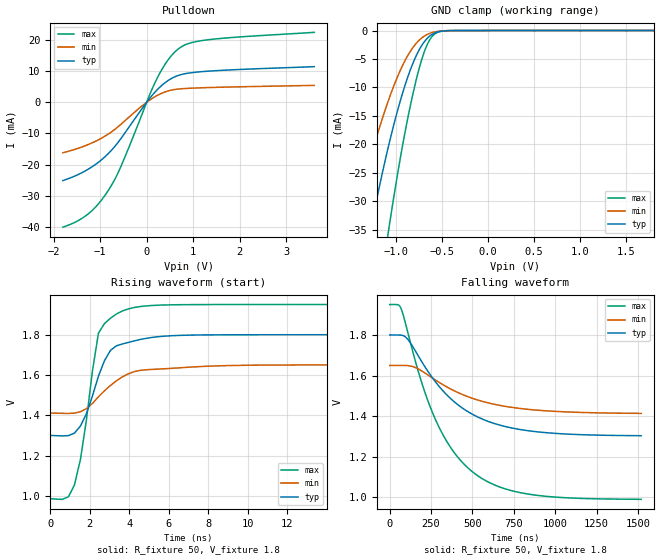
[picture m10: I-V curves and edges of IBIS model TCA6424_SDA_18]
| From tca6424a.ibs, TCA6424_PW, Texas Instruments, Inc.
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[Model]   TCA6424_SDA_18
Model_type  I/O_open_drain
Vinl=0.495
Vinh=1.365
Enable   Active-Low
Vref =   0
Rref =   500
Cref =   50p
Vmeas =   0.9
| variable   typ   min   max
C_comp   2.96pF   1.98pF   3.46pF
| C_pulldown   1.94pF   0.84pF   2.69pF
| C_tri-state   2.96pF   1.98pF   3.46pF
[Temperature Range]   40   100   -40
| Ambient temperature   25   85   -40
[Voltage range]   1.8   1.65   1.95
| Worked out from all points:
|   slope of the pulldown table from 0 to 0.27 V, typ, clamps not added: 57.9 ohm
|   GND clamp passes 1 mA (typ) near -0.63 V on its own axis
|   rising waveform, R_fixture 50, V_fixture 1.8: 20-80 % time 1.12ns typ, 1.74ns min, 830ps max; typ from 1.3 V to 1.8 V
|   falling waveform, R_fixture 50, V_fixture 1.8: 20-80 % time 345ns typ, 388ns min, 301ns max; typ from 1.8 V to 1.3 V
[GND Clamp]
| TCA6424_SDA_18
|   Voltage   I(typ)   I(min)   I(max)
-1.8V     -85.16mA   -58.96mA   -129.6mA
-1.475V   -52.78mA   -35.15mA   -83.81mA
-1.275V   -35.24mA   -22.59mA   -58.03mA
-1.075V   -20.18mA   -12.16mA   -35mA
-965mV    -13.27mA   -7.581mA   -23.93mA
-860mV    -7.809mA   -4.179mA   -14.77mA
-760mV    -3.889mA   -1.957mA   -7.626mA
-675mV    -1.704mA   -847.1uA   -3.151mA
-630mV    -976uA     -500.7uA   -1.642mA
-585mV    -504.4uA   -278.7uA   -738.2uA
-455mV    -43.99uA   -33.6uA    -41.78uA
1.8V      210pA      670.3pA    74.56pA
[Pulldown]
| TCA6424_SDA_18
|   Voltage   I(typ)   I(min)   I(max)
-1.8V     -25.1mA    -16.18mA   -40.03mA
-1.255V   -21.44mA   -13.54mA   -35.78mA
-1.045V   -19.33mA   -12.1mA    -32.72mA
-825mV    -16.46mA   -10.19mA   -28.27mA
-550mV    -11.56mA   -7.016mA   -20.47mA
60mV      1.174mA    652.4uA    2.253mA
215mV     3.846mA    2.097mA    7.413mA
445mV     6.827mA    3.573mA    13.29mA
680mV     8.622mA    4.255mA    17.11mA
920mV     9.403mA    4.495mA    18.95mA
1.315V    9.977mA    4.717mA    20.05mA
3.6V      11.43mA    5.425mA    22.44mA
[Ramp]
| TCA6424_SDA_18
| variable   typ   min   max
dV/dt_r   0.30/1.10E-09   0.14/1.74E-09   0.58/8.06E-10
dV/dt_f   0.30/3.45E-07   0.14/3.88E-07   0.58/3.01E-07
R_load = 50
[Rising Waveform]
| TCA6424_SDA_18
R_fixture =   50
C_fixture =   0
L_fixture =   0
V_fixture =   1.8
V_fixture_min = 1.65
V_fixture_max = 1.95
|   Time   V(typ)   V(min)   V(max)
0s        1.302V     1.412V     988.6mV
917ps     1.299V     1.409V     995.1mV
1.221ns   1.312V     1.411V     1.054V
1.525ns   1.346V     1.417V     1.18V
2.437ns   1.594V     1.492V     1.808V
2.741ns   1.671V     1.522V     1.855V
3.045ns   1.722V     1.548V     1.882V
3.653ns   1.754V     1.591V     1.918V
7.301ns   1.798V     1.64V      1.95V
1.52us    1.8V       1.65V      1.95V
[Falling Waveform]
| TCA6424_SDA_18
R_fixture =   50
C_fixture =   0
L_fixture =   0
V_fixture =   1.8
V_fixture_min = 1.65
V_fixture_max = 1.95
|   Time   V(typ)   V(min)   V(max)
0s        1.8V       1.65V      1.95V
69.01ns   1.8V       1.65V      1.929V
112.8ns   1.775V     1.649V     1.802V
198.2ns   1.663V     1.621V     1.553V
302.8ns   1.543V     1.565V     1.338V
398.5ns   1.465V     1.522V     1.211V
508.6ns   1.406V     1.486V     1.12V
652.1ns   1.359V     1.456V     1.055V
839.3ns   1.328V     1.434V     1.016V
1.52us    1.304V     1.414V     990.2mV
